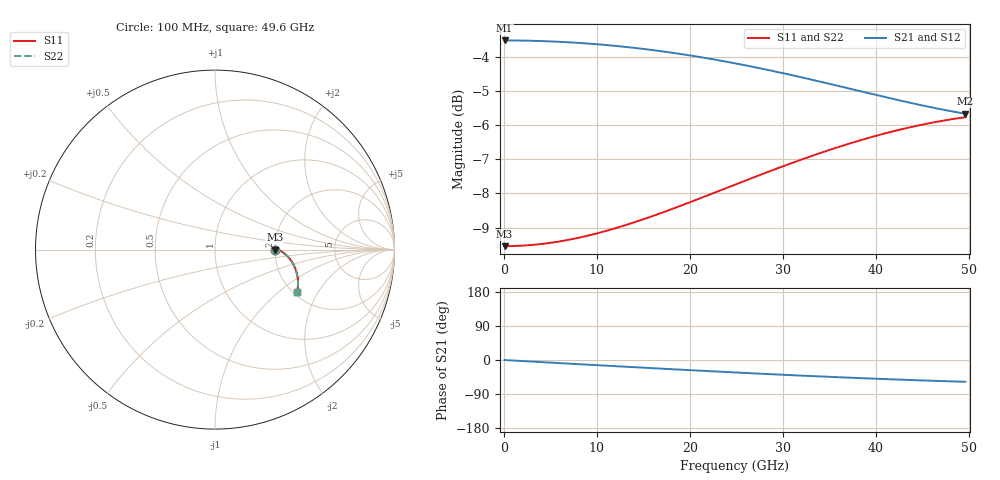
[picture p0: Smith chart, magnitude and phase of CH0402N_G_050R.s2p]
# GHz S RI R 50
! S-Parameters data
! Freq  reS11  imS11  reS21  imS21  reS12  imS12  reS22  imS22
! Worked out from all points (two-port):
!   100 points, 100 MHz to 49.6 GHz, reference 50 ohm
!   highest |S21| = -3.52 dB at 100 MHz (marker M1); lowest = -5.7 dB at 49.6 GHz (marker M2)
!   |S21| within 3 dB of the highest: start of sweep to end of sweep
!   lowest |S11| = -9.5 dB at 100 MHz (marker M3), VSWR 2.00, Z = 100 + j0.00471 ohm
!   |S11| at or under -10 dB: nowhere
!   |S22| runs from -9.5 to -5.8 dB; largest |S21 - S12| = 0
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0.1  0.3333 2.09e-05  0.6667 -0.00159  0.6667 -0.00159  0.3333 2.09e-05
2.1  0.334 0.000409  0.6655 -0.0334  0.6655 -0.0334  0.334 0.000409
4.1  0.3359 0.000626  0.6621 -0.065  0.6621 -0.065  0.3359 0.000626
6.1  0.3389 0.000514  0.6565 -0.0961  0.6565 -0.0961  0.3389 0.000514
8.6  0.3443 -0.000325  0.6466 -0.1341  0.6466 -0.1341  0.3443 -0.000325
10.6  0.3497 -0.00174  0.6365 -0.1636  0.6365 -0.1636  0.3497 -0.00174
12.6  0.3561 -0.00395  0.6245 -0.192  0.6245 -0.192  0.3561 -0.00395
14.6  0.3633 -0.0071  0.6107 -0.2193  0.6107 -0.2193  0.3633 -0.0071
16.6  0.3713 -0.0113  0.5953 -0.2451  0.5953 -0.2451  0.3713 -0.0113
19.1  0.3819 -0.0181  0.5741 -0.2753  0.5741 -0.2753  0.3819 -0.0181
21.1  0.3909 -0.025  0.5557 -0.2976  0.5557 -0.2976  0.3909 -0.025
23.1  0.4 -0.0332  0.5363 -0.3181  0.5363 -0.3181  0.4 -0.0332
25.1  0.4091 -0.0426  0.5161 -0.3369  0.5161 -0.3369  0.4091 -0.0426
27.1  0.4181 -0.0534  0.4952 -0.3539  0.4952 -0.3539  0.4181 -0.0534
29.1  0.4267 -0.0654  0.474 -0.369  0.474 -0.369  0.4267 -0.0654
31.1  0.4347 -0.0787  0.4527 -0.3823  0.4527 -0.3823  0.4347 -0.0787
33.1  0.4421 -0.0932  0.4313 -0.3938  0.4313 -0.3938  0.4421 -0.0932
37.1  0.4539 -0.1251  0.3896 -0.412  0.3896 -0.412  0.4539 -0.1251
39.6  0.4589 -0.1467  0.3647 -0.4204  0.3647 -0.4204  0.4589 -0.1467
41.6  0.4614 -0.1646  0.3457 -0.4258  0.3457 -0.4258  0.4614 -0.1646
45.6  0.4621 -0.2012  0.3105 -0.4337  0.3105 -0.4337  0.4621 -0.2012
49.6  0.4569 -0.2371  0.2796 -0.4394  0.2796 -0.4394  0.4569 -0.2371
